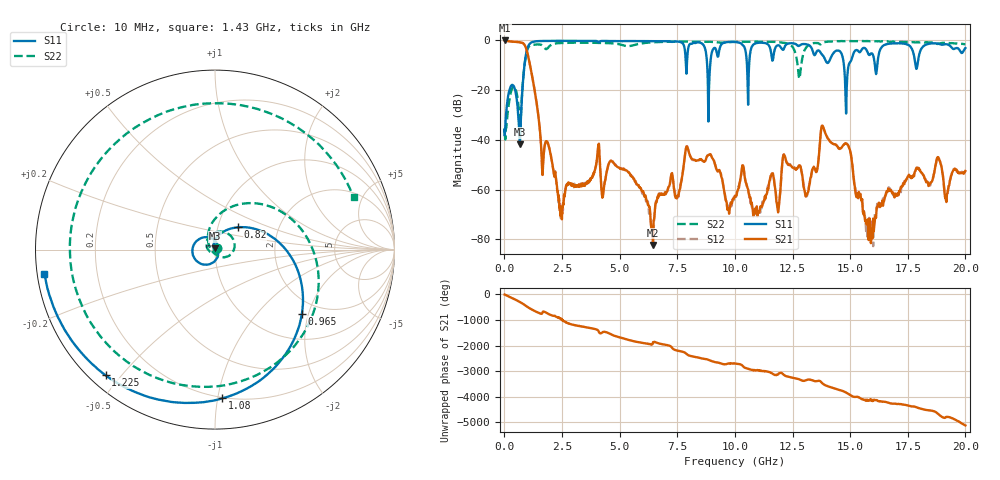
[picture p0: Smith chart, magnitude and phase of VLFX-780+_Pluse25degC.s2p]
! Mini-Circuits
! S2P DATA File Format
! Type: LOW PASS FILTER
! Model: VLFX-780+
! All S Parameters are in dB deg format
! TEST CONDITIONS: INPUT POWER = 0 dBm @ Temperature = +25 deg C
# MHz S DB R 50
!FREQ  MAG(S11)PHS(S11)MAG(S21)PHS(S21)MAG(S12)PHS(S12)MAG(S22)PHS(S22)
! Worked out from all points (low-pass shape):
!   1293 points, 10 MHz to 20 GHz, reference 50 ohm
!   highest |S21| = -0.07 dB at 10 MHz (marker M1); lowest = -82.3 dB at 6.45 GHz (marker M2)
!   |S21| within 3 dB of the highest: start of sweep to 935.7 MHz
!   lowest |S11| = -41.8 dB at 670 MHz (marker M3), VSWR 1.02, Z = 50.2 + j0.8 ohm
!   |S11| at or under -10 dB: start of sweep to 872 MHz; 8.798 GHz to 8.928 GHz (130.5 MHz wide, 1.47 % of centre); 14.73 GHz to 14.94 GHz (208 MHz wide, 1.4 % of centre)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
!   |S22| runs from -39.9 to -0.3 dB; largest |S21 - S12| = 0.0023
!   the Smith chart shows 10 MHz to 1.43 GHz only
!   S11 on the Smith chart (normalised r, x): 10 MHz: 1.02, +0.02; 820 MHz: 1.24, +0.32; 965 MHz: 1.61, -1.82; 1.08 GHz: 0.19, -1.03; 1.225 GHz: 0.05, -0.46; 1.43 GHz: 0.02, -0.07
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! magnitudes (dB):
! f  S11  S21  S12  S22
! 10 MHz  -38.1  -0.1  -0.1  -38.0
! 360 MHz  -18.0  -0.6  -0.6  -19.0
! 670 MHz  -41.8  -0.8  -0.8  -33.1
! 820 MHz  -15.0  -1.3  -1.3  -15.0
! 965 MHz  -4.4  -3.9  -3.9  -4.8
! 1.08 GHz  -1.6  -8.5  -8.5  -2.4
! 1.225 GHz  -0.7  -15.4  -15.4  -1.8
! 1.43 GHz  -0.4  -27.2  -27.2  -1.7
! 1.65 GHz  -0.3  -53.9  -54.0  -2.2
! 1.885 GHz  -0.3  -41.4  -41.3  -3.1
! 2.45 GHz  -0.2  -69.6  -71.5  -1.1
! 3.35 GHz  -0.2  -57.8  -58.4  -0.9
! 4.7 GHz  -0.3  -48.8  -48.6  -1.2
! 6.45 GHz  -0.4  -82.3  -76.5  -0.8
! 6.675 GHz  -0.4  -63.2  -62.1  -0.7
! 7.975 GHz  -3.2  -43.9  -44.0  -0.5
! 10.03 GHz  -0.7  -62.7  -62.4  -0.6
! 13.35 GHz  -3.6  -52.3  -52.2  -1.3
! 13.88 GHz  -6.9  -36.1  -36.1  -0.8
! 15.82 GHz  -5.9  -74.8  -71.4  -0.4
! 16.68 GHz  -1.4  -60.6  -59.1  -0.5
! 20 GHz  -3.1  -52.5  -52.5  -1.6
